TYPE LstGas :
STRUCT
	ToleranceMode:STRING;			//'Value' or 'Percent'
	ToleranceDelayTime:INT;	
	
	Gas1: INT;
	Gas1WarningRange:INT;
	Gas1AlarmRange:INT;
	
	Gas2: INT;
	Gas2WarningRange:INT;
	Gas2AlarmRange:INT;
	
	Gas3: INT;
	Gas3WarningRange:INT;
	Gas3AlarmRange:INT;
	
	Gas4: INT;
	Gas4WarningRange:INT;
	Gas4AlarmRange:INT;
	
	Gas5: INT;
	Gas5WarningRange:INT;
	Gas5AlarmRange:INT;
	
	Gas6: INT;
	Gas6WarningRange:INT;
	Gas6AlarmRange:INT;
	
	Gas7: INT;
	Gas7WarningRange:INT;
	Gas7AlarmRange:INT;
	
	Gas8: INT;
	Gas8WarningRange:INT;
	Gas8AlarmRange:INT;
	
	Gas9: INT;
	Gas9WarningRange:INT;
	Gas9AlarmRange:INT;
	
	
	(*GasEnableRamp: BOOL;
	Gas1Target: INT;
	Gas2Target: INT;
	Gas3Target: INT;
	Gas4Target: INT;
	Gas5Target: INT;
	Gas6Target: INT;
	Gas7Target: INT;
	Gas8Target: INT;
	//GasFlowRatie: INT;*)
END_STRUCT
END_TYPE
